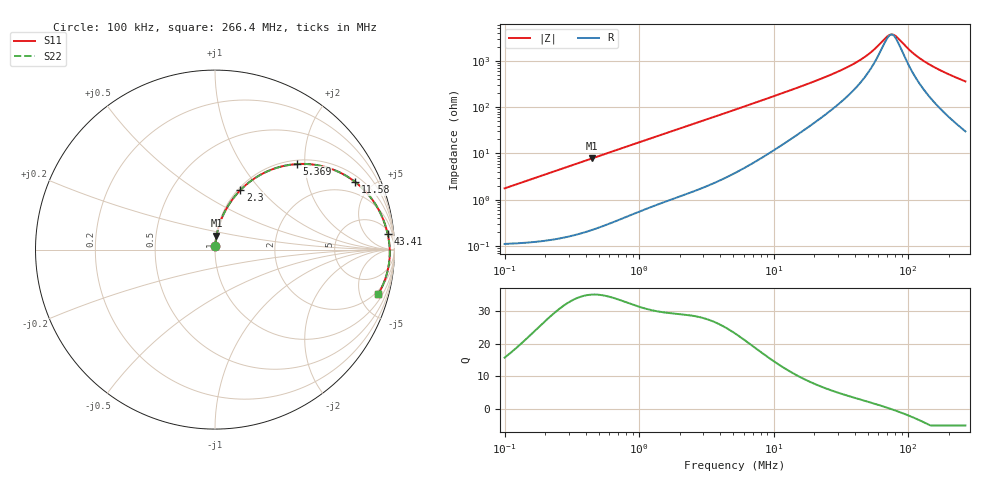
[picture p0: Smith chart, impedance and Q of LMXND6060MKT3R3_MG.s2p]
! LMXND6060MKT3R3_MG  S-PARAMETER MODEL  ( General Type )
! Model Generated by TAIYO YUDEN Corporation (http://www.ty-top.com)
! Version 1.0
! TAIYO YUDEN Control No. 191025NI43SB-FBB
! Copyright(c) 2019 TAIYO YUDEN CO.,LTD. All Rights Reserved.
! Product Description (link to TY-COMPAS)
! https://ds.yuden.co.jp/TYCOMPAS/or/detail?pn=LMXND6060MKT3R3NMG&u=M
! Products Name : Inductors
! Characteristics :
!  Inductance : 3.3 uH , SRF(min) : 42 MHz , DC Resistance(max) : 0.126 Ohm
!  Rated Current : Saturation :1800 mA , Temp Rise : 1700 mA
!  Case Size : 6.0 x 6.0 / 0.236 x 0.236 [mm/inch] , Thickness : 1.2 / 0.047 [mm/inch]
!  (Conditions: Temperature = 25 degC , DC Bias Current/Voltage = 0A / 0V)
! External Node Assignments :
!  1  o---GGG---o  2
! GND o---------o GND
! Frequency Range : 0.1MHz  -  266.375554MHz  [ 402 STEP ]
# MHz S RI R 50
! Freq[MHz].  S11 Real  S11 Imag  S21 Real  S21 Imag  S12 Real  S12 Imag  S22 Real  S22 Imag
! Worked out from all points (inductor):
!   401 points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, 100 kHz to 266.4 MHz, reference 50 ohm
!   read as one part in series: L = 2.8 uH near 104 kHz
!   highest Q = 35.1 at 447.6 kHz (marker M1), where L = 2.79 uH
!   self-resonance near 75.04 MHz
!   S11 on the Smith chart (normalised r, x): 100 kHz: 1.00, +0.04; 2.3 MHz: 1.03, +0.78; 5.369 MHz: 1.08, +1.82; 11.58 MHz: 1.31, +3.97; 43.41 MHz: 7, +19; 266.4 MHz: 1.60, -7.14
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0.1  0.00142 0.0175  0.9986 -0.0175  0.9986 -0.0175  0.00142 0.0175
0.374775  0.00618 0.0652  0.9938 -0.0652  0.9938 -0.0652  0.00618 0.0652
0.447552  0.0083 0.0776  0.9917 -0.0776  0.9917 -0.0776  0.0083 0.0776
0.808641  0.0234 0.1368  0.9766 -0.1368  0.9766 -0.1368  0.0234 0.1368
1.404561  0.062 0.225  0.938 -0.225  0.938 -0.225  0.062 0.225
2.299503  0.142 0.3322  0.858 -0.3322  0.858 -0.3322  0.142 0.3322
3.411212  0.2595 0.4203  0.7405 -0.4203  0.7405 -0.4203  0.2595 0.4203
5.26394  0.4467 0.4759  0.5533 -0.4759  0.5533 -0.4759  0.4467 0.4759
5.368768  0.4561 0.4766  0.5439 -0.4766  0.5439 -0.4766  0.4561 0.4766
7.656352  0.6233 0.4578  0.3767 -0.4578  0.3767 -0.4578  0.6233 0.4578
11.58405  0.7814 0.3766  0.2186 -0.3766  0.2186 -0.3766  0.7814 0.3766
19.34272  0.8959 0.2496  0.1041 -0.2496  0.1041 -0.2496  0.8959 0.2496
31.04897  0.9448 0.1477  0.0552 -0.1477  0.0552 -0.1477  0.9448 0.1477
43.41409  0.962 0.0876  0.038 -0.0876  0.038 -0.0876  0.962 0.0876
53.93017  0.9686 0.0521  0.0314 -0.0521  0.0314 -0.0521  0.9686 0.0521
72.49162  0.9733 0.00546  0.0267 -0.00546  0.0267 -0.00546  0.9733 0.00546
76.90933  0.9737 -0.00388  0.0263 0.00388  0.0263 0.00388  0.9737 -0.00388
81.59625  0.9738 -0.0133  0.0262 0.0133  0.0262 0.0133  0.9738 -0.0133
107.5381  0.9718 -0.0586  0.0282 0.0586  0.0282 0.0586  0.9718 -0.0586
138.9604  0.9649 -0.1045  0.0351 0.1045  0.0351 0.1045  0.9649 -0.1045
190.507  0.9469 -0.1684  0.0531 0.1684  0.0531 0.1684  0.9469 -0.1684
266.3756  0.91 -0.2473  0.09 0.2473  0.09 0.2473  0.91 -0.2473
